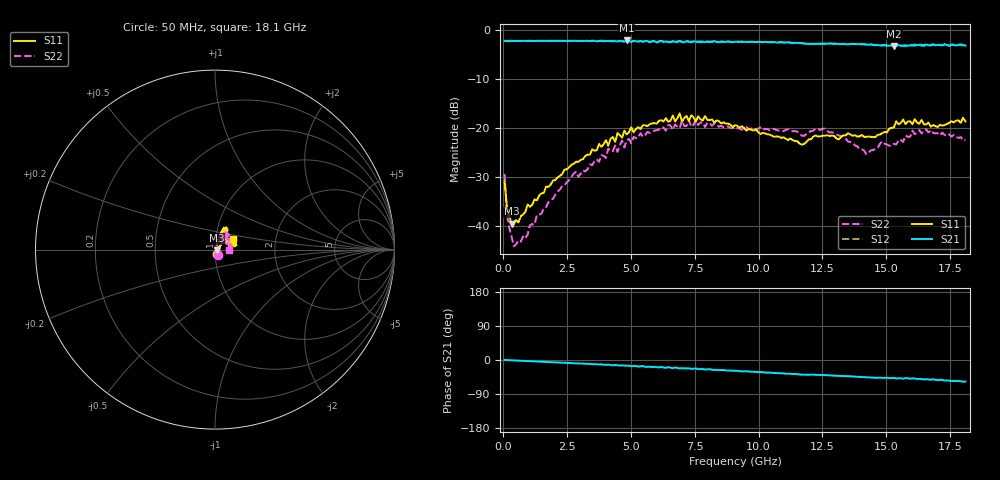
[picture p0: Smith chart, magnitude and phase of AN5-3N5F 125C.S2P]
! Network Analyzer HP8720D.06.14 Serial No. US36140669
! 27 Jun 2005  11:32:56
! Frequency  S11  S21  S12  S22
# HZ  S  DB R 50
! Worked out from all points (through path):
!   201 points, 50 MHz to 18.1 GHz, reference 50 ohm
!   highest |S21| = -2.18 dB at 4.833 GHz (marker M1); lowest = -3.3 dB at 15.3 GHz (marker M2)
!   group delay of S21, straight-line fit = 8.75 ps
!   lowest |S11| = -39.5 dB at 320.8 MHz (marker M3), VSWR 1.02, Z = 51 - j0.296 ohm
!   |S11| at or under -10 dB: start of sweep to end of sweep
!   |S22| runs from -44.1 to -18.4 dB; largest |S21 - S12| = 0.028
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5e7  -30.92 -61.8  -2.26 0.1  -2.29 0.4  -29.43 -57.7
1.4025e8  -36.14 -46.5  -2.32 -0.2  -2.31 -0.2  -37.56 -58.2
3.2075e8  -39.52 -15.9  -2.25 -0.7  -2.28 -0.6  -42.16 -27.9
4.11e8  -39.16 -9.6  -2.30 -1.2  -2.29 -1.2  -44.12 -15.9
8.6225e8  -37.12 18.6  -2.28 -2.4  -2.29 -2.4  -42.55 40.8
1.3135e9  -34.77 29.4  -2.26 -3.9  -2.28 -3.8  -37.73 43.7
3.1185e9  -26.36 44.5  -2.27 -9.3  -2.30 -9.6  -28.69 70.3
4.83325e9  -21.33 59.1  -2.18 -15.0  -2.31 -15.3  -22.44 61.8
6.09675e9  -18.56 59.4  -2.39 -19.4  -2.31 -19.2  -20.37 60.4
6.909e9  -17.05 63.1  -2.26 -22.3  -2.32 -21.1  -20.04 55.7
6.99925e9  -18.71 62.1  -2.44 -21.3  -2.57 -22.6  -18.49 57.0
7.54075e9  -18.75 61.1  -2.41 -22.3  -2.32 -24.3  -18.37 57.6
9.075e9  -19.46 68.1  -2.44 -28.4  -2.42 -28.6  -20.00 39.9
1.169225e10  -23.43 54.3  -2.75 -38.6  -2.76 -38.6  -21.60 39.4
1.21435e10  -21.76 51.6  -2.89 -38.6  -2.84 -38.8  -20.56 47.4
1.331675e10  -21.50 35.8  -2.91 -42.5  -2.92 -42.6  -21.78 41.8
1.421925e10  -21.83 15.3  -3.03 -45.3  -3.01 -45.4  -25.37 42.3
1.512175e10  -20.13 19.7  -3.25 -47.8  -3.13 -47.6  -23.64 32.6
1.530225e10  -19.90 16.9  -3.31 -47.4  -3.21 -48.8  -23.26 37.0
1.566325e10  -18.30 14.9  -3.28 -49.1  -3.18 -47.8  -22.85 26.5
1.656575e10  -19.31 11.5  -3.01 -50.7  -3.01 -51.6  -20.36 14.2
1.81e10  -18.68 29.0  -3.23 -56.7  -3.27 -57.2  -22.41 -0.0
